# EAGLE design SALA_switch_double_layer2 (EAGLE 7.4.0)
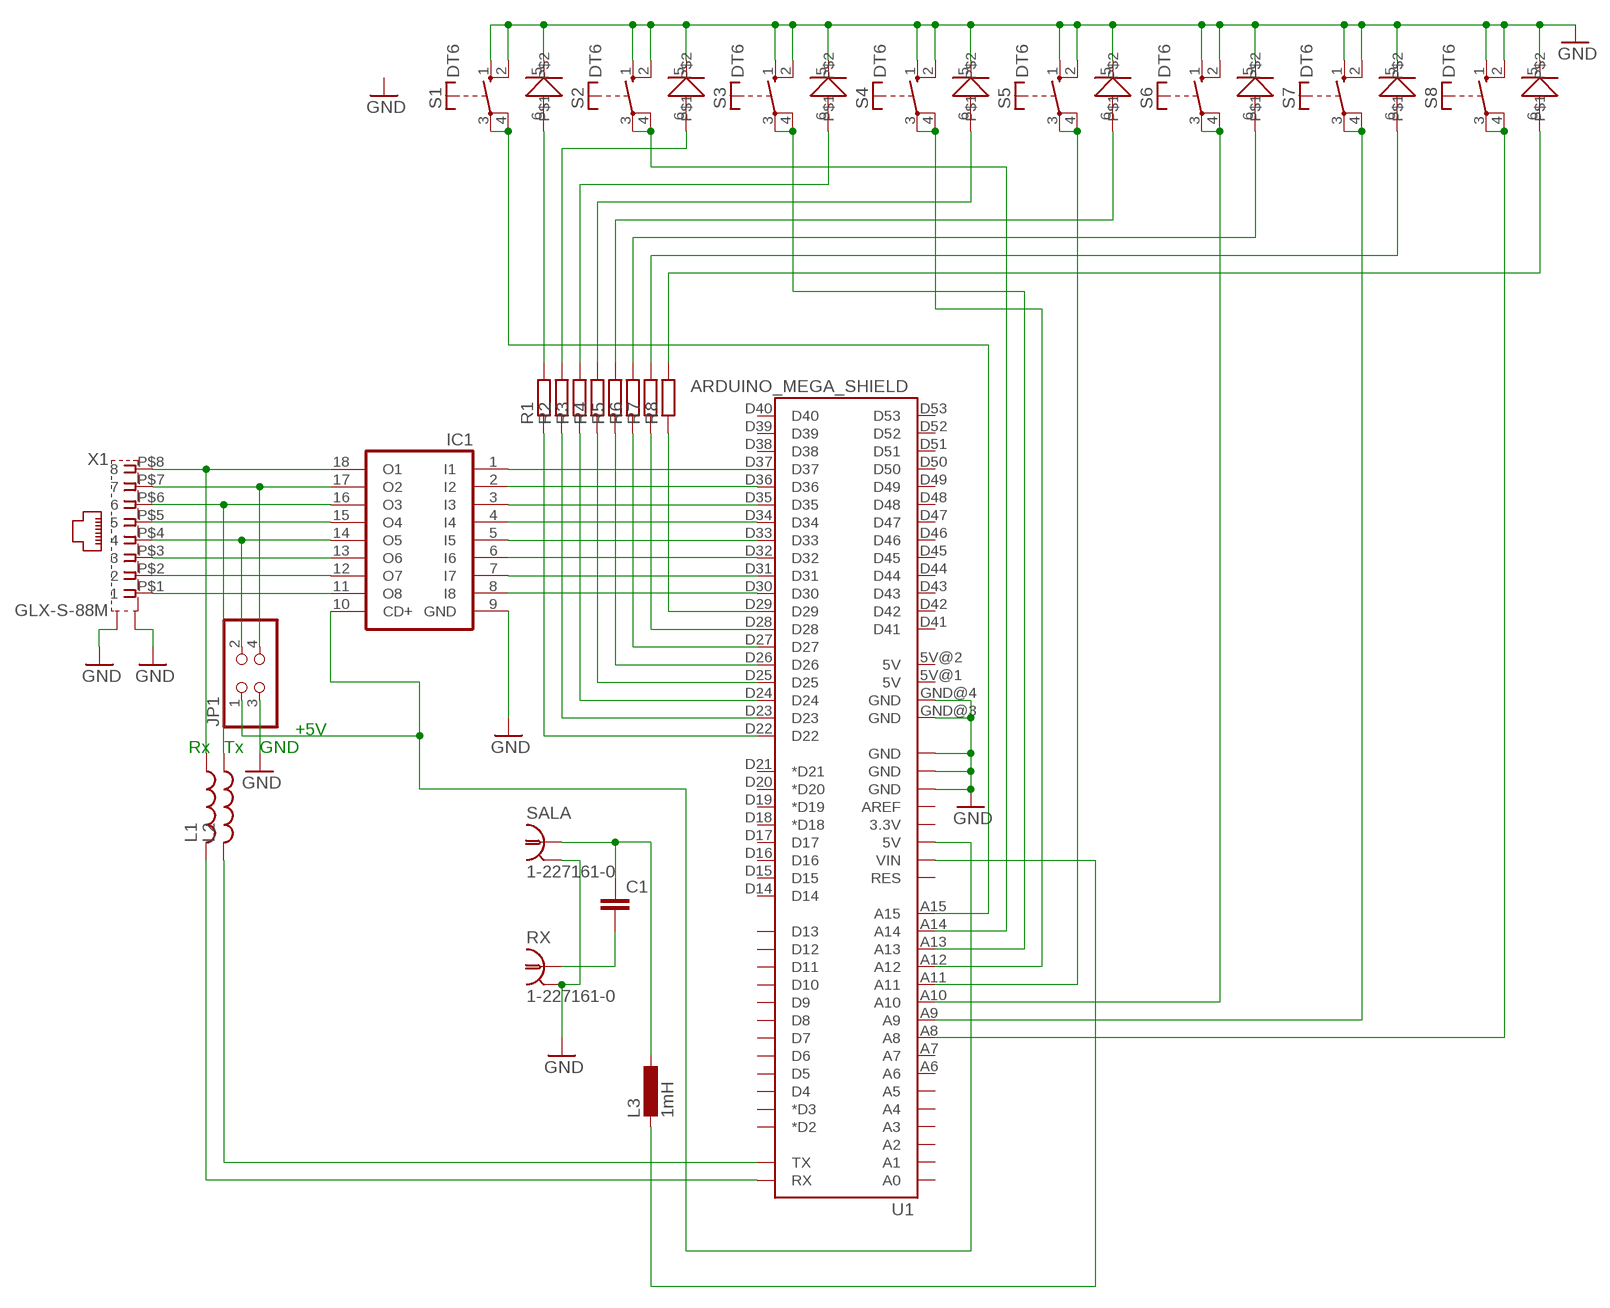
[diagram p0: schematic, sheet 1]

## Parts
C1  C-EU025-024X044  [C025-024X044]
IC1  ULN2803A  [DIL18]
JP1  PINHD-2X2  [2X02]
L1  L-USL2012C  [L2012C]
L2  L-USL2012C  [L2012C]
L3  1mH  L-EU0207/10  [0207/10]
R1  R-EU_R0805  [R0805]
R2  R-EU_R0805  [R0805]
R3  R-EU_R0805  [R0805]
R4  R-EU_R0805  [R0805]
R5  R-EU_R0805  [R0805]
R6  R-EU_R0805  [R0805]
R7  R-EU_R0805  [R0805]
R8  R-EU_R0805  [R0805]
RX  1-227161-0  [AMP_227161]
S1  DT6  [DT6]
S2  DT6  [DT6]
S3  DT6  [DT6]
S4  DT6  [DT6]
S5  DT6  [DT6]
S6  DT6  [DT6]
S7  DT6  [DT6]
S8  DT6  [DT6]
SALA  1-227161-0  [AMP_227161]
U1  ARDUINO_MEGA_SHIELD  [ARDUINO_MEGA_SHIELD]
X1  GLX-S-88M  [GLX-S-88M]

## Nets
GND: IC1.9(GND) JP1.3 RX.2 S1.1(S) S1.2(S) S1.5 S2.1(S) S2.2(S) S2.5 S3.1(S) S3.2(S) S3.5 S4.1(S) S4.2(S) S4.5 S5.1(S) S5.2(S) S5.5 S6.1(S) S6.2(S) S6.5 S7.1(S) S7.2(S) S7.5 S8.1(S) S8.2(S) S8.5 SALA.2 U1.GND@0(GND) U1.GND@1(GND) U1.GND@2(GND) U1.GND@3(GND) U1.GND@4(GND) X1.P$9(S1) X1.P$10(S2)
N$1: R1.2 S1.6
N$2: R2.2 S2.6
N$3: R3.2 S3.6
N$4: R4.2 S4.6
N$5: R1.1 U1.D22
N$6: R5.2 S5.6
N$7: R6.2 S6.6
N$8: R7.2 S7.6
N$9: R2.1 U1.D23
N$10: R3.1 U1.D24
N$11: R4.1 U1.D25
N$12: R5.1 U1.D26
N$13: R6.1 U1.D27
N$14: R7.1 U1.D28
N$15: R8.1 U1.D29
N$16: R8.2 S8.6
N$17: S1.3(P) S1.4(P) U1.A15
N$18: S2.3(P) S2.4(P) U1.A14
N$19: S3.3(P) S3.4(P) U1.A13
N$20: S4.3(P) S4.4(P) U1.A12
N$21: S5.3(P) S5.4(P) U1.A11
N$22: S6.3(P) S6.4(P) U1.A10
N$23: S7.3(P) S7.4(P) U1.A9
N$24: S8.3(P) S8.4(P) U1.A8
N$25: IC1.18(O1) L1.1 X1.P$8
N$26: L3.2 U1.VIN
N$27: IC1.17(O2) JP1.4 X1.P$7
N$28: IC1.16(O3) L2.1 X1.P$6
N$29: IC1.15(O4) X1.P$5
N$30: IC1.14(O5) JP1.2 X1.P$4
N$31: IC1.13(O6) X1.P$3
N$32: IC1.12(O7) X1.P$2
N$33: IC1.11(O8) X1.P$1
N$34: IC1.1(I1) U1.D37
N$35: IC1.2(I2) U1.D36
N$36: IC1.3(I3) U1.D35
N$37: IC1.4(I4) U1.D34
N$38: IC1.5(I5) U1.D33
N$39: IC1.6(I6) U1.D32
N$40: IC1.7(I7) U1.D31
N$41: IC1.8(I8) U1.D30
N$42: IC1.10(CD+) JP1.1 U1.5V@0(5V)
N$43: C1.1 L3.1 SALA.1
N$44: C1.2 RX.1
N$46: L2.2 U1.TX
N$47: L1.2 U1.RX
Unconnected: U1.3.3V U1.5V@1(5V) U1.5V@2(5V) U1.A0 U1.A1 U1.A2 U1.A3 U1.A4 U1.A5 U1.A6 U1.A7 U1.AREF U1.D2(*D2) U1.D3(*D3) U1.D4 U1.D5 U1.D6 U1.D7 U1.D8 U1.D9 U1.D10 U1.D11 U1.D12 U1.D13 U1.D14 U1.D15 U1.D16 U1.D17 U1.D18(*D18) U1.D19(*D19) U1.D20(*D20) U1.D21(*D21) U1.D38 U1.D39 U1.D40 U1.D41 U1.D42 U1.D43 U1.D44 U1.D45 U1.D46 U1.D47 U1.D48 U1.D49 U1.D50 U1.D51 U1.D52 U1.D53 U1.RES

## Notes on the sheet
- +5V
- Rx | Tx | GND

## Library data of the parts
C1 = resistor:C-EU: CAPACITOR, European symbol
IC1 = uln-udn:ULN2803A: DRIVER ARRAY
JP1 = pinhead:PINHD-2X2: PIN HEADER
L1 L2 = resistor:L-US: INDUCTOR, American symbol
L3 = resistor:L-EU: INDUCTOR, European symbol
R1-R8 = resistor:R-EU_: RESISTOR, European symbol
RX SALA = con-coax:?227161*: JACK, RIGHT ANGLE, 50 OHM, PCB, BNC; MF: TYCO ELECTRONICS; MPN: 1-227161; OC_FARNELL: unknown; OC_NEWARK: 33B3200
S1-S8 = switch-misc:DT: ITT SWITCH
U1 = RepRapjr:ARDUINO_MEGA_SHIELD
X1 = con-kycon:GLX-S-88M: Mod. Jack, Right Angle, 8 posiotion, 8 contatcs RJ45 Source: GLX-S-88M.pdf; OC_FARNELL: unknown; OC_NEWARK: unknown

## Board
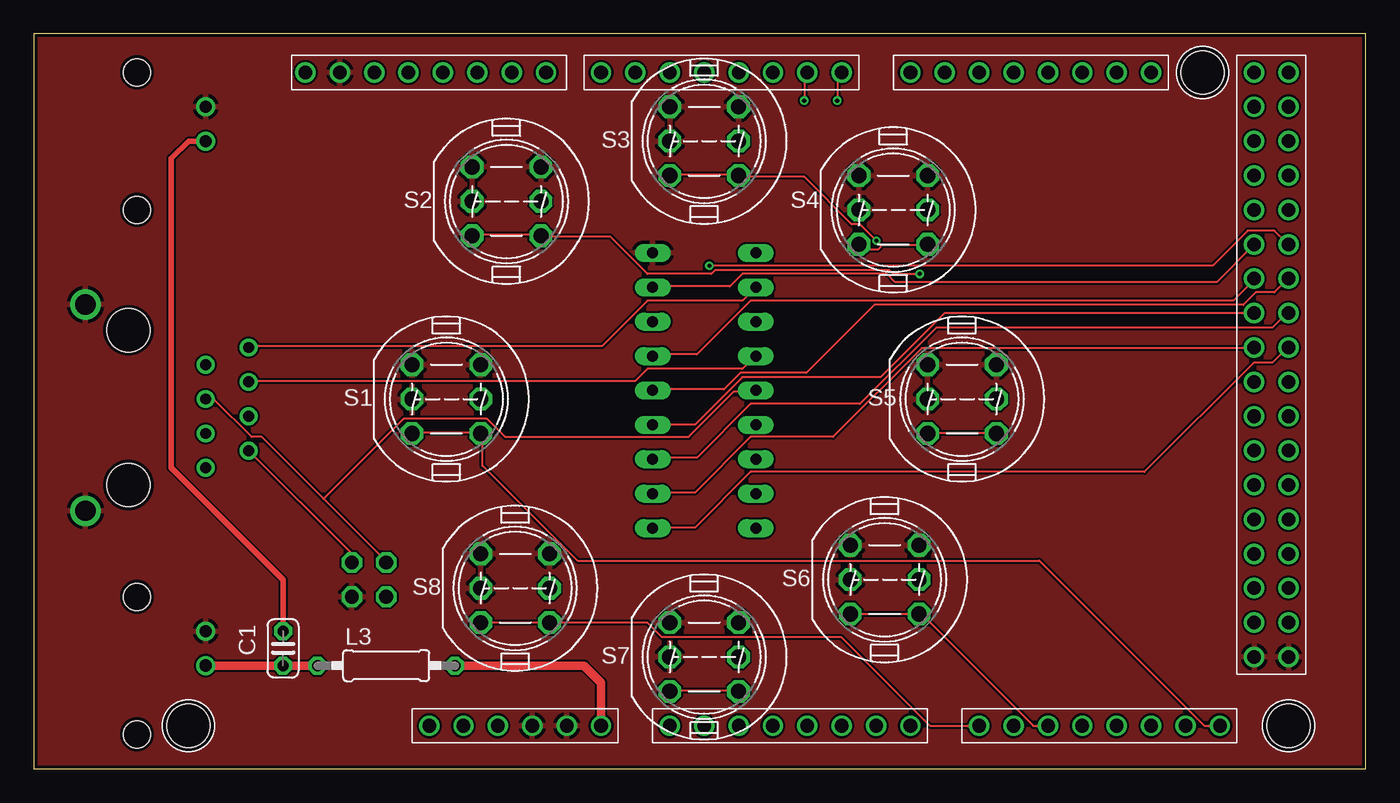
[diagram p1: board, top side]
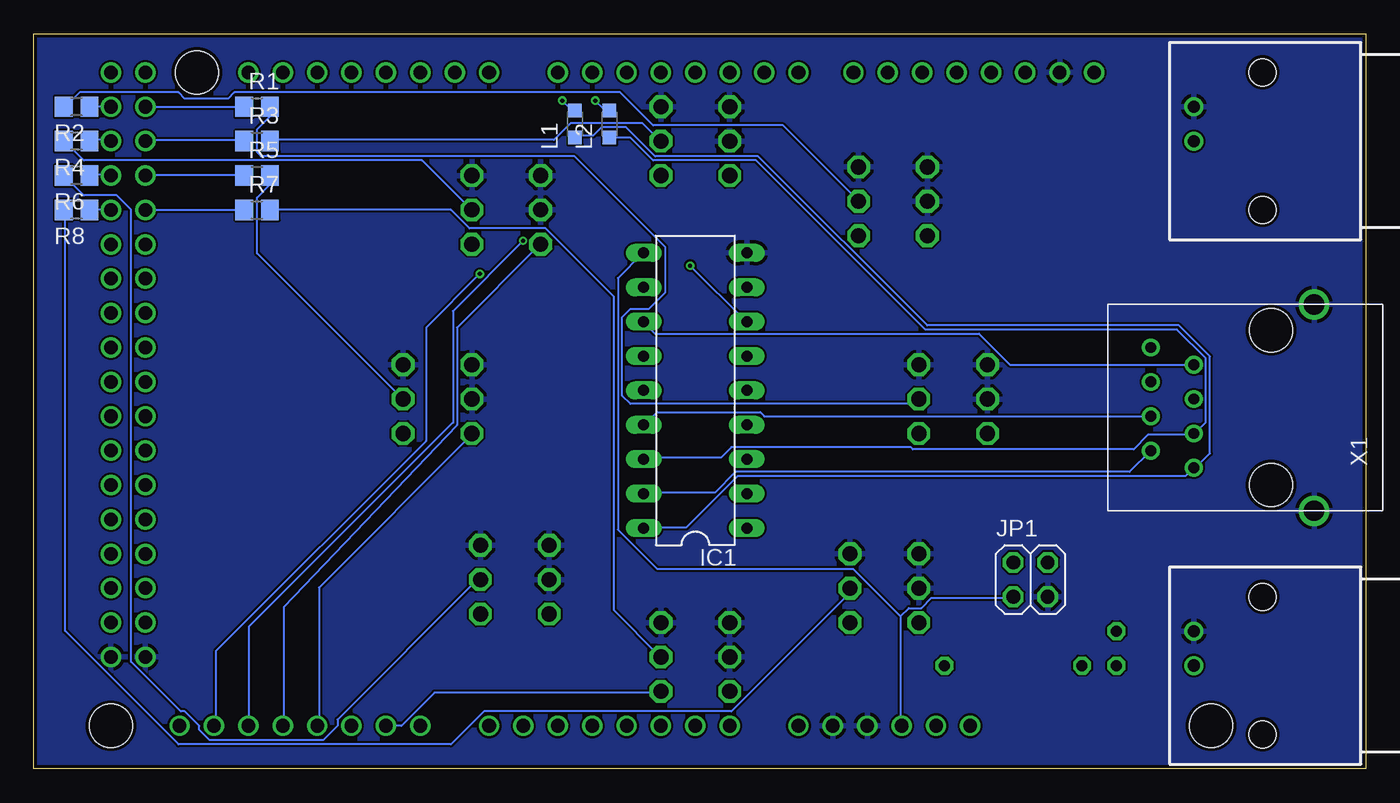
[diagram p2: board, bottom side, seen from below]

Size 98.41 x 54.28 mm. Coordinates in mm from the lower left corner, seen from the top.
Outline: 0,0 98.41,0 98.41,54.28 0,54.28 0,0
Copper layers (1*16): Top 0.035mm / dielectric 1.5mm / Bottom 0.035mm
Design rules "SeeedStudio_2layer_DRU_no_angle_20140221": minimum track width 6mil, minimum drill 12mil, track to track 6mil, track to pad 6mil, pad to pad 6mil, via to via 6mil, smd to smd 0mil, copper to edge 10mil, drill to drill 10mil, minimum pad ring 10mil, minimum via ring 6mil, stop-mask expansion 2mil, vias tented up to drill 100mil, thermal gap 10mil

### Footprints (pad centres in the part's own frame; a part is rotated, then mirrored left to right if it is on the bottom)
C025-024X044 = drill 0.813 octagon: 1 -1.27,0; 2 1.27,0
DIL18 = drill 0.813 long: 1 -10.16,-3.81; 2 -7.62,-3.81; 3 -5.08,-3.81; 4 -2.54,-3.81; 5 0,-3.81; 6 2.54,-3.81; 7 5.08,-3.81; 8 7.62,-3.81; 9 10.16,-3.81; 10 10.16,3.81; 11 7.62,3.81; 12 5.08,3.81; 13 2.54,3.81; 14 0,3.81; 15 -2.54,3.81; 16 -5.08,3.81; 17 -7.62,3.81; 18 -10.16,3.81
2X02 = drill 1.016 octagon: 1 -1.27,-1.27; 2 -1.27,1.27; 3 1.27,-1.27; 4 1.27,1.27
L2012C = smd 1 x 1: 1 -1,0; 2 1,0
0207/10 = drill 0.813 octagon: 1 -5.08,0; 2 5.08,0
R0805 = smd 1.3 x 1.5: 1 -0.95,0; 2 0.95,0
AMP_227161 = drill 0.9 pad 1.27: 1 0,-5.08; 2 -2.54,-5.08 | hole 2: -5.08,0; 5.08,0
DT6 = drill 1.118 octagon: 1 -2.54,2.54; 2 2.54,2.54; 3 2.54,-2.54; 4 -2.54,-2.54; 5 -2.54,0; 6 2.54,0
ARDUINO_MEGA_SHIELD = drill 1 pad 1.422: 3.3V 50.8,26.67; 5V@0 50.8,29.21; 5V@1 2.54,85.09; 5V@2 2.54,87.63; A0 50.8,41.91; A1 50.8,44.45; A2 50.8,46.99; A3 50.8,49.53; A4 50.8,52.07; A5 50.8,54.61; A6 50.8,57.15; A7 50.8,59.69; A8 50.8,64.77; A9 50.8,67.31; A10 50.8,69.85; A11 50.8,72.39; A12 50.8,74.93; A13 50.8,77.47; A14 50.8,80.01; A15 50.8,82.55; AREF 2.54,14.986; D2 2.54,49.53; D3 2.54,46.99; D4 2.54,44.45; D5 2.54,41.91; D6 2.54,39.37; D7 2.54,36.83; D8 2.54,32.766; D9 2.54,30.226; D10 2.54,27.686; D11 2.54,25.146; D12 2.54,22.606; D13 2.54,20.066; D14 2.54,59.69; D15 2.54,62.23; D16 2.54,64.77; D17 2.54,67.31; D18 2.54,69.85; D19 2.54,72.39; D20 2.54,74.93; D21 2.54,77.47; D22 5.08,85.09; D23 5.08,87.63; D24 7.62,85.09; D25 7.62,87.63; D26 10.16,85.09; D27 10.16,87.63; D28 12.7,85.09; D29 12.7,87.63; D30 15.24,85.09; D31 15.24,87.63; D32 17.78,85.09; D33 17.78,87.63; D34 20.32,85.09; D35 20.32,87.63; D36 22.86,85.09; D37 22.86,87.63; D38 25.4,85.09; D39 25.4,87.63; D40 27.94,85.09; D41 27.94,87.63; D42 30.48,85.09; D43 30.48,87.63; D44 33.02,85.09; D45 33.02,87.63; D46 35.56,85.09; D47 35.56,87.63; D48 38.1,85.09; D49 38.1,87.63; D50 40.64,85.09; D51 40.64,87.63; D52 43.18,85.09; D53 43.18,87.63; GND@0 50.8,31.75; GND@1 50.8,34.29; GND@2 2.54,17.526; GND@3 45.72,85.09; GND@4 45.72,87.63; RES 50.8,24.13; RX 2.54,54.61; TX 2.54,52.07; VIN 50.8,36.83 | hole 3.2: 2.54,81.28; 50.8,87.63; 50.8,6.35
GLX-S-88M = drill 0.8: P$1 4.445,3.175; P$2 3.175,0; P$3 1.905,3.175; P$4 0.635,0; P$5 -0.635,3.175; P$6 -1.905,0; P$7 -3.175,3.175; P$8 -4.445,0 | drill 1.5: P$9 -7.62,-8.89; P$10 7.62,-8.89 | hole 3.2: -5.715,-5.715; 5.715,-5.715

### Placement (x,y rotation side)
C1  18.41,8.89 90 top
IC1  49.53,27.94 90 bottom
JP1  24.77,13.97 0 bottom
L1  58.42,47.62 90 bottom
L2  55.88,47.62 90 bottom
L3  26.04,7.62 0 top
R1  81.92,48.9 0 bottom
R2  95.25,48.9 180 bottom
R3  81.92,46.36 0 bottom
R4  95.25,46.36 180 bottom
R5  81.92,43.82 0 bottom
R6  95.25,43.82 180 bottom
R7  81.92,41.28 0 bottom
R8  95.25,41.28 180 bottom
RX  7.62,46.36 270 bottom
S1  30.48,27.31 0 top
S2  34.93,41.91 0 top
S3  49.53,46.36 0 top
S4  63.5,41.28 0 top
S5  68.58,27.31 0 top
S6  62.86,13.97 0 top
S7  49.53,8.25 0 top
S8  35.56,13.34 0 top
SALA  7.62,7.62 270 bottom
U1  5.08,53.98 270 top
X1  12.7,26.67 90 bottom

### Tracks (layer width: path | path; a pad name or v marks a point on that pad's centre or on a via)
GND
  Top 0.152: S5.5 66.06,27.25 66.12,27.38 | S5.1 66.06,29.85 65.96,29.77
  pour Bottom: 0,54.61 98.42,54.61 98.42,0 0,0
  pour Top: 0,54.61 98.42,54.61 98.42,0 0,0
N$1
  Bottom 0.152: R1.2 81,48.9 81,48.13 81.92,47.22 81.92,45.54 81.61,45.24 58.45,45.24 51.74,38.53 51.74,35.18 52.96,33.96 54.33,33.96 54.94,33.35 54.94,27.56 54.33,26.95 33.45,26.95 33.15,27.25 S1.6
N$2
  Bottom 0.152: R2.2 96.09,48.9 95.02,49.96 87.71,49.96 87.25,49.51 84.05,49.51 83.59,49.96 55.09,49.96 52.65,47.52 43.05,47.52 37.57,42.04 S2.6
N$3
  Bottom 0.152: R3.2 80.85,46.46 59.97,46.46 58.75,47.68 53.42,47.68 52.2,46.46 S3.6
N$4
  Bottom 0.152: R4.2 96.09,46.3 94.72,44.93 69.72,44.93 66.06,41.28 S4.6
N$5
  Bottom 0.152: U1.D22 R1.1
N$6
  Bottom 0.152: R5.2 81,43.71 81,43.1 81.92,42.19 81.92,38.08 71.25,27.41 S5.6
N$7
  Bottom 0.152: R6.2 96.09,43.71 94.72,42.34 92.28,42.34 91.21,41.28 91.21,7.9 87.55,4.24 87.25,4.24 86.18,3.18 86.18,2.87 85.42,2.11 77.04,2.11 75.97,3.18 75.97,3.63 65.76,13.84 65.46,13.84 S6.6
N$8
  Bottom 0.152: R7.2 67.59,41.28 66.22,39.9 60.58,39.9 55.55,34.87 55.55,11.71 52.2,8.36 S7.6
N$9
  Bottom 0.152: U1.D23 R2.1
N$10
  Bottom 0.152: R3.1 82.98,46.46 90.14,46.46 U1.D24
N$11
  Bottom 0.152: 94.87,46.46 R4.1 94.26,46.46 92.73,46.46 U1.D25
N$12
  Bottom 0.152: R5.1 82.98,43.87 90.14,43.87 U1.D26
N$13
  Bottom 0.152: R6.1 94.26,43.87 92.73,43.87 U1.D27
N$14
  Bottom 0.152: U1.D28 R7.1
N$15
  Bottom 0.152: U1.D29 R8.1
N$16
  Bottom 0.152: R8.2 96.09,41.28 96.09,10.18 87.71,1.8 67.59,1.8 65.15,4.24 46.86,4.24 38.18,12.93 38.18,13.23 S8.6
N$17
  Top 0.152: U1.A15 86.49,3.18 74.3,15.37 40.16,15.37 33.15,22.38 33.15,24.66 S1.3 33,24.82 27.97,24.82 S1.4
N$18  (via drill 0.3)
  Top 0.152: v65.46,36.55 63.48,36.55 63.17,36.86 50.37,36.86 50.06,36.55 45.34,36.55 42.6,39.29 37.57,39.29 S2.3 | 37.41,39.29 S2.3 | S2.4 32.39,39.45 37.41,39.45 S2.3
  Bottom 0.152: v65.46,36.55 69.42,32.59 69.42,24.21 | 69.42,24.21 | 69.42,24.21 84.96,8.66 84.96,3.18 U1.A14
N$19  (via drill 0.3)
  Top 0.152: v62.25,38.99 61.04,40.21 60.43,40.21 56.92,43.71 52.2,43.71 S3.3 | 52.05,43.71 S3.3 | S3.4 47.02,43.87 52.05,43.87 S3.3
  Bottom 0.152: 67.44,25.58 67.44,33.81 v62.25,38.99 | 67.44,25.58 67.44,25.53 | 67.44,25.58 82.53,10.49 82.53,3.18 U1.A13
N$20
  Top 0.152: S4.3 65.91,38.68 62.71,38.68 62.41,38.38 61.34,38.38 61.04,38.68 S4.4
  Bottom 0.152: U1.A12 79.93,3.18 79.93,11.94 67.13,25.38 67.13,32.59 61.04,38.68 S4.4
N$21
  Top 0.152: S5.3 71.09,24.82 66.06,24.82 S5.4
  Bottom 0.152: U1.A11 77.34,3.18 77.34,13.39 66.06,24.66 S5.4
N$22
  Top 0.152: U1.A10 73.84,3.18 65.46,11.56 S6.3 65.3,11.41 60.43,11.41 S6.4
N$23
  Top 0.152: S7.4 47.02,5.77 52.05,5.77 S7.3
  Bottom 0.152: U1.A9 71.25,3.18 68.81,5.61 52.2,5.61 S7.3
N$24
  Top 0.152: U1.A8 66.22,3.18 59.67,9.73 46.41,9.73 45.34,10.79 S8.3 S8.4
N$25
  Bottom 0.152: IC1.18 53.26,17.81 50.22,17.81 46.41,21.61 13.34,21.61 12.73,22.23 X1.P$8 12.57,22.23 11.51,23.29 11.51,30.46 13.79,32.74 32.39,32.74 44.88,45.24 52.5,45.24 54.64,47.37 56.46,47.37 57.07,46.76 58.29,46.76 L1.1
N$26
  Top 0.61: U1.VIN 41.91,6.35 40.64,7.62 L3.2
N$27
  Top 0.152: X1.P$7 23.39,15.98 23.39,15.37 JP1.4
  Bottom 0.152: X1.P$7 17.45,21.92 46.56,21.92 48.08,20.4 53.26,20.4 IC1.17
N$28
  Bottom 0.152: IC1.16 53.26,22.99 47.62,22.99 46.86,23.75 33.6,23.75 33.45,23.6 17.15,23.6 16.08,24.66 12.73,24.66 X1.P$6 12.57,24.82 11.81,25.58 11.81,30.3 13.95,32.44 32.54,32.44 45.03,44.93 52.65,44.93 54.33,46.61 55.86,46.61 L2.1
N$29
  Bottom 0.152: X1.P$5 44.42,26.04 44.73,26.34 52.35,26.34 53.26,25.43 IC1.15
N$30
  Top 0.152: 21.41,19.94 25.98,15.37 JP1.2 | 21.41,19.94 16.84,24.51 16.08,24.51 13.34,27.25 12.73,27.25 X1.P$4 | 21.41,19.94 27.36,25.88 33.45,25.88 34.82,24.51 48.39,24.51 51.74,27.86 53.26,27.86 IC1.14
N$31
  Top 0.152: X1.P$3 15.93,28.63 44.42,28.63 45.34,29.54 52.35,29.54 53.26,30.46 IC1.13
N$32
  Bottom 0.152: IC1.12 53.26,32.89 52.5,32.13 28.58,32.13 26.29,29.85 X1.P$2
N$33
  Top 0.152: IC1.11 52.35,34.57 45.34,34.57 41.99,31.22 15.93,31.22 X1.P$1
N$34
  Top 0.152: IC1.1 45.8,17.81 48.84,17.81 52.96,21.92 82.07,21.92 90.14,30 91.52,30 92.58,31.06 U1.D37
N$35
  Top 0.152: IC1.2 45.8,20.4 48.84,20.4 52.96,24.51 59.06,24.51 65.61,31.06 90.14,31.06 U1.D36
N$36
  Top 0.152: IC1.3 45.8,22.99 49,22.99 52.96,26.95 61.04,26.95 66.67,32.59 91.52,32.59 92.58,33.66 U1.D35
N$37
  Top 0.152: U1.D34 67.28,33.66 62.56,28.93 52.35,28.93 48.84,25.43 45.8,25.43 IC1.4
N$38
  Top 0.152: IC1.5 45.8,28.02 50.98,28.02 52.2,29.24 57.07,29.24 62.1,34.27 89.38,34.27 90.3,35.18 91.67,35.18 92.58,36.09 U1.D33
N$39
  Top 0.152: IC1.6 45.8,30.61 49,30.61 52.96,34.57 88.62,34.57 90.14,36.09 U1.D32
N$40  (via drill 0.3)
  Top 0.152: v49.91,37.16 87.1,37.16 89.69,39.75 91.67,39.75 92.58,38.84 U1.D31
  Bottom 0.152: v49.91,37.16 45.8,33.05 IC1.7
N$41
  Top 0.152: IC1.8 45.8,35.64 51.44,35.64 52.35,36.55 63.02,36.55 63.63,35.94 87.4,35.94 90.14,38.68 U1.D30
N$42
  Bottom 0.152: 34.37,11.25 34.37,3.18 U1.5V@0 | 34.37,11.25 37.87,14.76 52.35,14.76 55.25,17.65 55.25,36.25 53.42,38.08 IC1.10 | 34.37,11.25 33.76,11.86 32.84,11.86 32.08,12.62 26.14,12.62 JP1.1
N$43
  Top 0.61: L3.1 C1.1 SALA.1
N$44
  Top 0.406: RX.1 11.43,46.36 10.16,45.09 10.16,22.23 18.41,13.97 C1.2
N$46  (via drill 0.3)
  Top 0.152: v56.92,49.35 56.92,51.18 57.07,51.33 U1.TX
  Bottom 0.152: v56.92,49.35 56.31,48.74 56.01,48.74 L2.2
N$47  (via drill 0.3)
  Top 0.152: v59.36,49.35 59.36,51.03 59.67,51.33 U1.RX
  Bottom 0.152: v59.36,49.35 58.75,48.74 58.45,48.74 L1.2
